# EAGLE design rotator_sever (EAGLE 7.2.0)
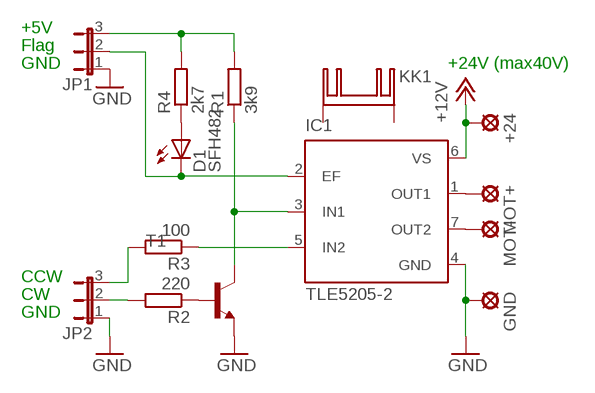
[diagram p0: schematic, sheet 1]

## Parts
+24  +24V  LSP13  [LSP13]
D1  SFH482  [SFH482]
GND  LSP13  [LSP13]
IC1  TLE5205-2  [P-TO220-7-11]
JP1  JP2E  [JP2]
JP2  JP2E  [JP2]
KK1  SK129-PAD  [SK129]
MOT+  LSP13  [LSP13]
MOT-  LSP13  [LSP13]
R1  3k9  R-EU_0207/10  [0207/10]
R2  220  R-EU_0207/10  [0207/10]
R3  100  R-EU_0207/10  [0207/10]
R4  2k7  R-EU_0207/10  [0207/10]
T1  2N5550-NPN-TO92-CBE  [TO92-CBE]

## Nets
+12V: +24.MP IC1.6(VS)
GND: GND.MP IC1.4(GND) JP1.1 JP2.1 T1.E
N$1: IC1.1(OUT1) MOT+.MP
N$2: IC1.7(OUT2) MOT-.MP
N$3: JP2.2 R2.2
N$4: IC1.3(IN1) R1.1 T1.C
N$5: JP2.3 R3.2
N$6: R2.1 T1.B
N$7: JP1.3 R1.2 R4.2
N$8: IC1.5(IN2) R3.1
N$9: D1.A R4.1
N$10: D1.K(C) IC1.2(EF) JP1.2
Unconnected: KK1.A2,5(K) KK1.B2,5(K)

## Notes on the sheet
- +5V
- Flag
- GND | +24V (max40V)
- CCW
- CW
- GND

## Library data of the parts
+24 GND MOT+ MOT- = solpad:LSP13: SOLDER PAD
D1 = led:SFH482: IR LED
IC1 = infineon:TLE5205-2: 5-A H-Bridge for DC-Motor Applications Source: http://www.infineon.com .. tle5205-2.pdf; OC_FARNELL: unknown; OC_NEWARK: unknown
JP1 JP2 = jumper:JP2E: JUMPER
KK1 = heatsink:SK129-PAD: HEATSINK
R1-R4 = rcl:R-EU_: RESISTOR, European symbol
T1 = transistor:*-NPN-: NPN Transistror BF959 corrected 2008.03.06

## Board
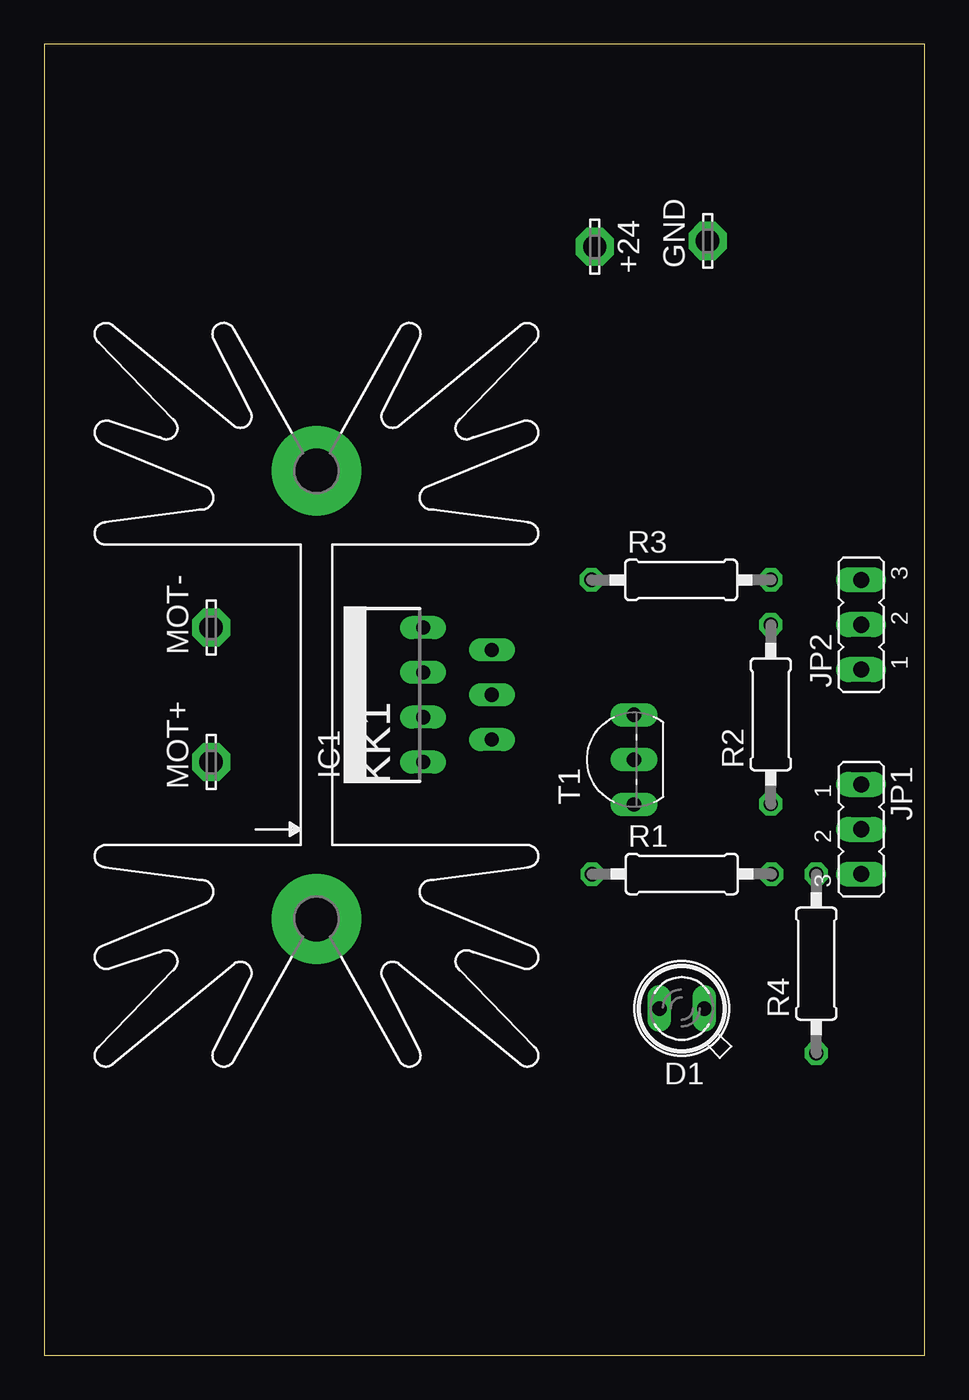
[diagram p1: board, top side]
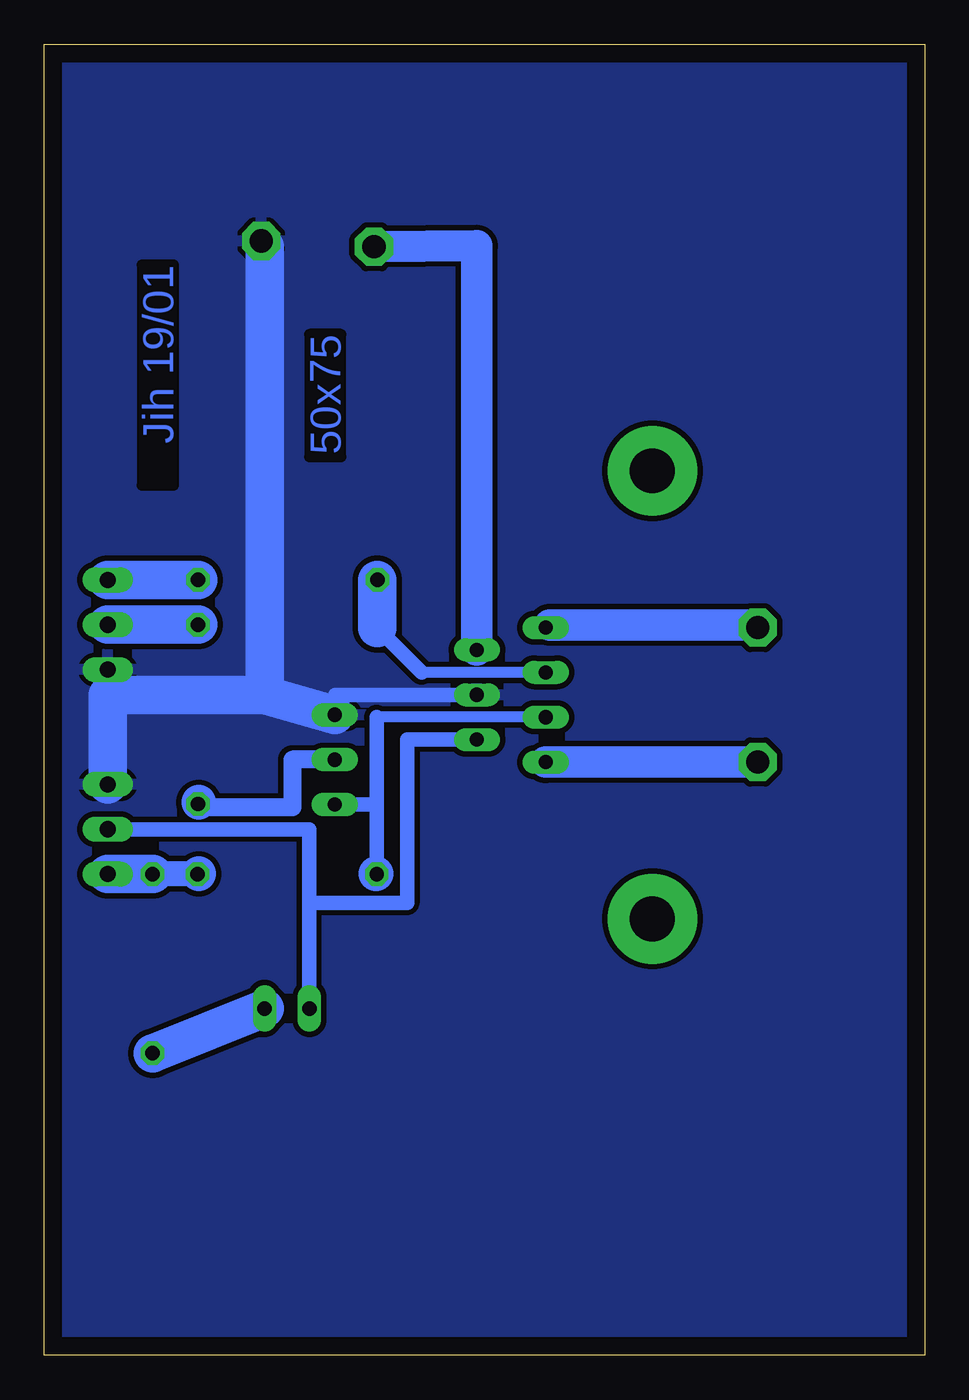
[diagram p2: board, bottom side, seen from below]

Size 49.9 x 74.33 mm. Coordinates in mm from the lower left corner, seen from the top.
Outline: 49.9,0 49.9,74.33 0,74.33 0,0 49.9,0
Copper layers (1*16): Top 0.035mm / dielectric 1.5mm / Bottom 0.035mm
Design rules "default": minimum track width 10mil, minimum drill 24mil, track to track 8mil, track to pad 8mil, pad to pad 8mil, via to via 8mil, smd to smd 8mil, copper to edge 40mil, drill to drill 8mil, minimum pad ring 10mil, minimum via ring 8mil, stop-mask expansion 4mil, vias tented up to drill 0mil, thermal gap 10mil

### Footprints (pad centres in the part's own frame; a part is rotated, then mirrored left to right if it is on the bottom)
LSP13 = drill 1.321 pad 2.159 octagon: MP 0,0
SFH482 = drill 0.813 long: A -1.27,0; K 1.27,0
P-TO220-7-11 = drill 0.8 pad 1.2 long: 1 -3.81,-1.85; 2 -2.54,-5.75; 3 -1.27,-1.85; 4 0,-5.75; 5 1.27,-1.85; 6 2.54,-5.75; 7 3.81,-1.85
JP2 = drill 0.914 long: 1 -2.54,0; 2 0,0; 3 2.54,0
SK129 = drill 2.54 pad 5.08: A2,5 -12.7,-0.889; B2,5 12.7,-0.889
0207/10 = drill 0.813 octagon: 1 -5.08,0; 2 5.08,0
TO92-CBE = drill 0.813 long: B 0,0; C -2.54,0; E 2.54,0

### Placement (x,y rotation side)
+24  31.21,62.85 270 top
D1  36.13,19.67 180 top
GND  37.59,63.17 90 top
IC1  19.62,37.45 90 top
JP1  46.3,29.83 270 top
JP2  46.3,41.42 90 top
KK1  14.54,37.45 90 top
MOT+  9.46,33.64 90 top
MOT-  9.46,41.26 90 top
R1  36.13,27.29 0 top
R2  41.18,36.34 90 top
R3  36.1,43.96 0 top
R4  43.76,22.21 90 top
T1  33.43,33.77 90 top

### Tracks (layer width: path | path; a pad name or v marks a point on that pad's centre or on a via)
+12V
  Bottom 1.778: IC1.6 25.38,62.9 +24.MP
GND
  Bottom 0.254: 46.3,37.45 JP2.1
  Bottom 0.813: IC1.4 33.4,37.45 33.4,36.29
  Bottom 2.184: JP1.1 46.3,37.45 37.41,37.45 | T1.E 37.41,37.45 | GND.MP 37.41,62.85 37.41,37.45
  pour Bottom (isolate 0.305): -1.44,-1.31 -1.44,74.88 50.55,74.88 50.88,-0.98
N$1
  Bottom 1.778: MOT+.MP IC1.1
N$2
  Bottom 0.254: 21.25,41.41 IC1.7 | 9.59,41.41 MOT-.MP
  Bottom 1.778: 9.59,41.41 21.25,41.41
N$3
  Bottom 2.184: R2.2 JP2.2
N$4
  Bottom 0.61: IC1.3 31.05,36.18
  Bottom 0.813: 31.05,36.18 31.05,31.23 | 31.05,31.23 R1.1 | T1.C 31.05,31.23
N$5
  Bottom 2.184: R3.2 JP2.3
N$6
  Bottom 1.016: T1.B 35.84,33.77 35.84,31.07 41.18,31.07 R2.1
N$7
  Bottom 1.422: R1.2 R4.2
  Bottom 2.184: R4.2 JP1.3
N$8
  Bottom 0.61: IC1.5 28.52,38.72
  Bottom 0.813: 28.52,38.72 31.02,41.22
  Bottom 2.184: 31.02,41.22 R3.1
N$9
  Bottom 2.184: D1.A R4.1
N$10
  Bottom 0.813: IC1.2 29.33,34.91 29.33,25.66 34.87,25.66 | D1.K 34.87,25.66 | JP1.2 34.87,29.83 34.87,25.76 34.87,25.66
(copper drawn outside any net)
  shapes: Bottom circle x3

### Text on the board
Bottom: Jih 19/01 | 50x75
